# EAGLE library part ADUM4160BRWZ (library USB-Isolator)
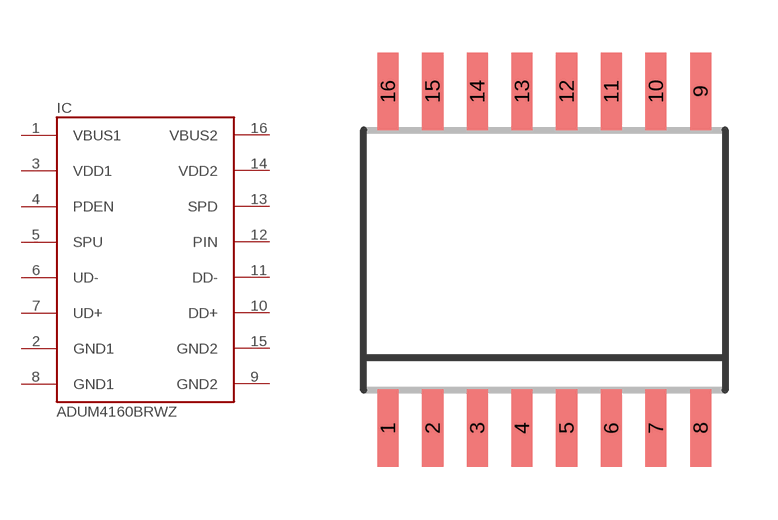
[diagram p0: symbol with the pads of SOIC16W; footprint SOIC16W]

Designator prefix IC

## ADUM4160BRWZ  [SOIC16W]
1  VBUS1  pwr
2  GND1  pwr
3  VDD1  pwr
4  PDEN
5  SPU
6  UD-
7  UD+
8  GND1  pwr
9  GND2  pwr
10  DD+
11  DD-
12  PIN
13  SPD
14  VDD2  pwr
15  GND2  pwr
16  VBUS2  pwr

## Footprint SOIC16W (pad centres in mm)
16-Lead SOIC (R) Package Source: http://www.analog.com/static/imported-files/data_sheets/AD745.pdf
smd 0.6 x 2.2: 1 -4.445,-4.775; 2 -3.175,-4.775; 3 -1.905,-4.775; 4 -0.635,-4.775; 5 0.635,-4.775; 6 1.905,-4.775; 7 3.175,-4.775; 8 4.445,-4.775; 9 4.445,4.8; 10 3.175,4.8; 11 1.905,4.8; 12 0.635,4.8; 13 -0.635,4.8; 14 -1.905,4.8; 15 -3.175,4.8; 16 -4.445,4.8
